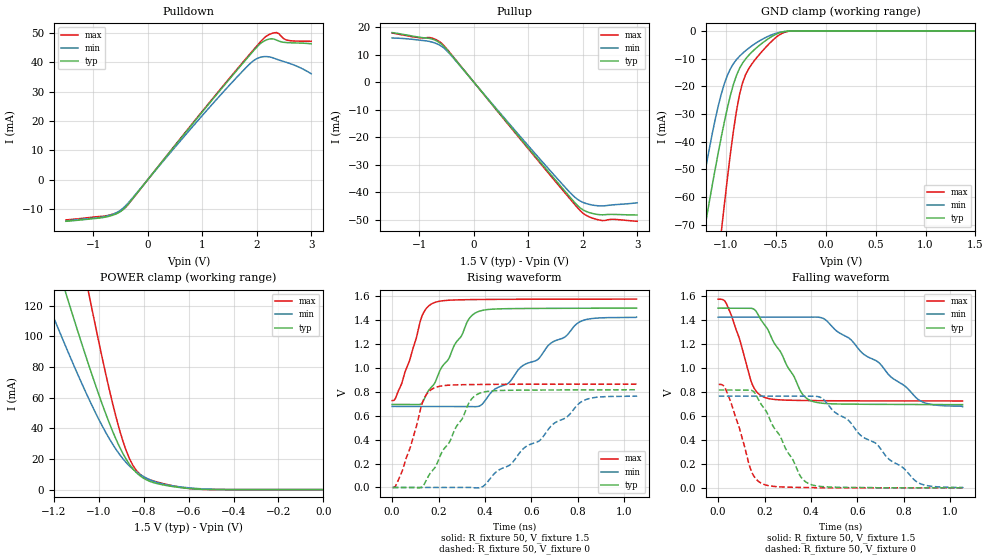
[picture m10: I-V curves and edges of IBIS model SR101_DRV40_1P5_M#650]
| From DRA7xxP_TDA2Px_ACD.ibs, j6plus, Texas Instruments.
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| Model based on original model for DDR_DIFFIOPB_H
|   Sub model SR101_DRV40_1P5
[model]   SR101_DRV40_1P5_M#650
|[Description]  [1.5V-I/O-X-X]
|   , ,
|[Input Load]
|[Output Drive]
|Voltage   1.5V
|Mode   I/O
Model_type   I/O
Polarity   Non-Inverting
Enable   Active-Low
Vinl =  0.65
Vinh =  0.85
Cref =  15.0000pF
Rref =  100.0000M
Vref =  0V
Vmeas =  0.75
C_comp   2p   2p   2p
[Model Spec]
Vinl   0.65   0.6125   0.6875
Vinh   0.85   0.8125   0.8875
[Receiver Thresholds]
Tslew_ac = 0.5n
Vth = 0.75
Vth_max = 0.7875
Vth_min = 0.675
Vinh_ac = 0.175
Vinh_dc = 0.1
Vinl_ac = -0.175
Vinl_dc = -0.1
[Temperature Range]   25   125   -40
[Voltage Range]   1.5   1.425   1.575
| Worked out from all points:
|   slope of the pulldown table from 0 to 0.225 V, typ, clamps not added: 43 ohm
|   slope of the pullup table from 0 to 0.225 V, typ, clamps not added: 41.7 ohm
|   GND clamp passes 1 mA (typ) near -0.48 V on its own axis
|   POWER clamp passes 1 mA (typ) near -0.62 V on its own axis
|   rising waveform, R_fixture 50, V_fixture 1.5: 20-80 % time 136ps typ, 308ps min, 78.1ps max; typ from 0.695 V to 1.5 V
|   rising waveform, R_fixture 50, V_fixture 0: 20-80 % time 135ps typ, 299ps min, 78ps max; typ from 0 V to 0.817 V
|   falling waveform, R_fixture 50, V_fixture 1.5: 20-80 % time 134ps typ, 278ps min, 77.5ps max; typ from 1.5 V to 0.695 V
|   falling waveform, R_fixture 50, V_fixture 0: 20-80 % time 135ps typ, 288ps min, 77.9ps max; typ from 0.817 V to 0 V
[POWER_clamp]
-1.5V     302.8mA    223.9mA    484.4mA
-1.242V   174.3mA    127.3mA    279.1mA
-1.136V   123.3mA    89.68mA    196.8mA
-1.045V   81.65mA    59.62mA    128.8mA
-1.03V    75mA       54.92mA    117.8mA
-939.4mV  38.44mA    29.91mA    56.84mA
-893.9mV  23.93mA    20.41mA    32.31mA
-848.5mV  13.61mA    13.43mA    15.91mA
-803mV    7.623mA    8.663mA    8.564mA
-712.1mV  3.022mA    3.561mA    3.877mA
-575.8mV  470.5uA    872uA      449uA
0V        112.6nA    435.6nA    613.8nA
[Pulldown]
-1.5V     -14.18mA   -14.05mA   -13.7mA
-727.3mV  -12.54mA   -12.27mA   -12.15mA
-545.5mV  -11.35mA   -10.95mA   -11.1mA
-409.1mV  -9.378mA   -8.925mA   -9.416mA
1.227V    28.16mA    26.58mA    28.43mA
1.818V    41.23mA    38.42mA    41.56mA
2V        45.11mA    41.2mA     45.49mA
2.182V    47.62mA    41.92mA    48.94mA
2.273V    47.99mA    41.65mA    49.78mA
2.364V    47.57mA    41.06mA    50.1mA
2.545V    46.7mA     39.96mA    47.58mA
3V        46.28mA    36.09mA    47.12mA
[Pullup]
-1.5V     17.97mA    16.01mA    17.82mA
-1V       16.28mA    15.23mA    16.1mA
-772.7mV  15.66mA    14.54mA    16.02mA
-590.9mV  13.75mA    12.97mA    14.08mA
-409.1mV  9.799mA    9.534mA    9.955mA
1.409V    -33.42mA   -32.26mA   -33.94mA
1.773V    -41.87mA   -40.19mA   -42.52mA
1.909V    -44.87mA   -42.6mA    -45.68mA
2.091V    -47.15mA   -44.23mA   -48.65mA
2.318V    -48.13mA   -44.93mA   -50.11mA
2.591V    -48.02mA   -44.49mA   -49.82mA
3V        -48.22mA   -43.8mA    -50.51mA
[GND_clamp]
-1.5V     -133.6mA   -115.7mA   -234.3mA
-1.288V   -87.29mA   -67.59mA   -156.8mA
-1.197V   -68.11mA   -48.64mA   -124.4mA
-1.045V   -38.25mA   -22.77mA   -72.51mA
-1.015V   -32.88mA   -19.1mA    -62.74mA
-954.5mV  -23.3mA    -13.72mA   -44.4mA
-863.6mV  -13.6mA    -9.192mA   -23.11mA
-803mV    -10.18mA   -7.193mA   -15.89mA
-681.8mV  -5.771mA   -4.027mA   -9.287mA
-500mV    -1.264mA   -914.7uA   -2.429mA
-348.5mV  -52.39uA   -75.11uA   -85.87uA
1.5V      112.6nA    528.1nA    514.5nA
[Ramp]
dV/dt_f 0.48371638/0.1344601n 0.44929255/0.27899089n 0.51008323/77.587251p
dV/dt_r 0.49174227/0.13539252n 0.46153752/0.30103568n 0.51970717/78.162105p
R_load = 50
[Rising Waveform]
R_fixture = 50
V_fixture = 1.5
V_fixture_min = 1.425
V_fixture_max = 1.575
0s        694.7mV    677.7mV    726.3mV
40.92ps   694mV      677.6mV    867.3mV
129.9ps   708.9mV    677.6mV    1.438V
178.6ps   858.2mV    677.7mV    1.543V
328ps     1.401V     676.8mV    1.571V
372.1ps   1.472V     678.6mV    1.572V
555.7ps   1.496V     1.009V     1.574V
626.7ps   1.497V     1.069V     1.574V
805.6ps   1.499V     1.382V     1.575V
1.053ns   1.5V       1.425V     1.575V
[Rising Waveform]
R_fixture = 50
V_fixture = 0
V_fixture_min = 0
V_fixture_max = 0
2.617ps   0V         0V         0V
43.65ps   0V         0V         137.9mV
134.3ps   15.11mV    0V         728.9mV
181.2ps   156.8mV    0V         832.2mV
332.5ps   712.7mV    0V         860.5mV
376.6ps   787.9mV    0V         861.5mV
571.4ps   814.1mV    334.9mV    863.4mV
636.5ps   814.9mV    394.4mV    863.6mV
819ps     816.1mV    721.2mV    863.9mV
1.055ns   817.1mV    766.1mV    864.1mV
[Falling Waveform]
R_fixture = 50
V_fixture = 1.5
V_fixture_min = 1.425
V_fixture_max = 1.575
0s        1.5V       1.425V     1.575V
37ps      1.5V       1.425V     1.532V
91.62ps   1.5V       1.425V     1.246V
144ps     1.499V     1.425V     877.9mV
195.5ps   1.373V     1.425V     758.8mV
357.2ps   799.6mV    1.425V     729.5mV
401.2ps   726mV      1.426V     728.5mV
461.8ps   704.2mV    1.404V     727.5mV
868.6ps   695.8mV    728.9mV    725.6mV
1.053ns   694.7mV    677.7mV    725.4mV
[Falling Waveform]
R_fixture = 50
V_fixture = 0
V_fixture_min = 0
V_fixture_max = 0
2.617ps   817.1mV    766.1mV    864.1mV
26.17ps   817.2mV    766.1mV    845.5mV
51.72ps   817.2mV    766.1mV    731.9mV
144.1ps   813.5mV    766.2mV    135mV
193.2ps   677.1mV    766.1mV    31.72mV
352.5ps   102.6mV    766mV      3.47mV
395.2ps   31.13mV    766.5mV    2.395mV
451.1ps   10.07mV    742.9mV    0V
857.4ps   0V         48.03mV    0V
1.055ns   0V         0V         0V
